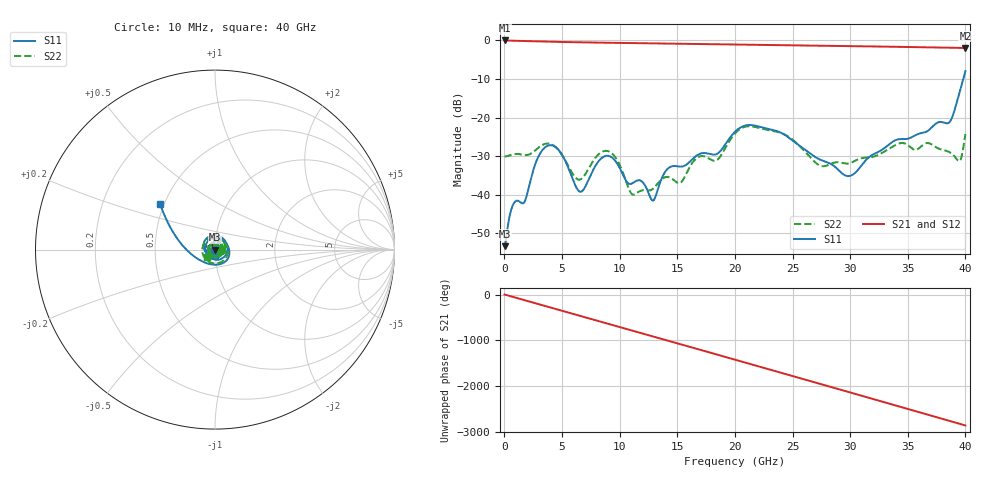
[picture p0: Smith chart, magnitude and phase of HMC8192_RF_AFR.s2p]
! Analog Devices, Inc.
! 1 Analog Way
! Wilmington, MA 01887
! http://www.analog.com
! Date:  2021-09-17 NN
! Board Name:  EVALHMC8192LG Revision A with HMC8192LG installed
! File Description:  Automatic Fixture Removal S-Parameters for RF Port connector and board loss de-embedding
! File Generation:  Calibrated Network Analyzer
! Chip Part Number:  HMC8192
! Chip Description:  Wideband IQ Mixer
! Chip Frequency:  20 to 42 GHz
! Chip Package:  LGA_CAV, 4 x 4 x 1.55 mm
! RF Port:  HMC8192LG removed and end of trace left open
! Note:
!  Analog Devices supplies this data as a sample of measured data at the evaluation board
!  ports for this product.  Your particular data for this product may vary.
!  Analog Devices reserves the right to change this data at anytime.
!  All lines below in this file are as is from the Network Analyzer.
!Agilent Technologies,N5245A,MY52451809,A.10.47.06
!Automatic Fixture Removal (AFR)
!Date: Friday, September 17, 2021 3:03:46 AM
!S2P File: Measurements: S11,S21,S12,S22:
# MHz S  RI  R 50
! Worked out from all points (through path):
!   4000 points, 10 MHz to 40 GHz, reference 50 ohm
!   highest |S21| = 0.00 dB at 10 MHz (marker M1); lowest = -1.9 dB at 40 GHz (marker M2)
!   group delay of S21, straight-line fit = 199 ps
!   lowest |S11| = -53.3 dB at 10 MHz (marker M3), VSWR 1.00, Z = 49.8 + j0.0141 ohm
!   |S11| at or under -10 dB: start of sweep to 39.81 GHz
!   |S22| runs from -39.9 to -22.2 dB; largest |S21 - S12| = 1.5e-15
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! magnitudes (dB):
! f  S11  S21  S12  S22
! 10 MHz  -53.3  0.0  0.0  -30.0
! 720 MHz  -42.7  -0.1  -0.1  -29.5
! 1.74 GHz  -41.8  -0.2  -0.2  -29.7
! 3.59 GHz  -27.5  -0.3  -0.3  -26.7
! 4.74 GHz  -28.5  -0.4  -0.4  -28.6
! 6.68 GHz  -39.1  -0.5  -0.5  -35.8
! 8.89 GHz  -29.9  -0.6  -0.6  -28.6
! 11.1 GHz  -37.0  -0.7  -0.7  -39.9
! 12.85 GHz  -41.5  -0.7  -0.7  -38.5
! 13.34 GHz  -38.3  -0.8  -0.8  -36.9
! 14.35 GHz  -32.8  -0.8  -0.8  -35.5
! 15.3 GHz  -32.7  -0.9  -0.9  -36.8
! 16.92 GHz  -29.4  -0.9  -0.9  -30.1
! 18.44 GHz  -29.4  -1.0  -1.0  -31.0
! 20.01 GHz  -23.6  -1.1  -1.1  -24.1
! 23.92 GHz  -23.8  -1.2  -1.2  -23.9
! 26.67 GHz  -29.6  -1.3  -1.3  -30.7
! 29.91 GHz  -35.1  -1.5  -1.5  -31.8
! 33.34 GHz  -27.0  -1.6  -1.6  -28.1
! 38.58 GHz  -21.3  -1.9  -1.9  -28.9
! 39.49 GHz  -13.5  -1.9  -1.9  -31.2
! 40 GHz  -7.9  -1.9  -1.9  -24.3
